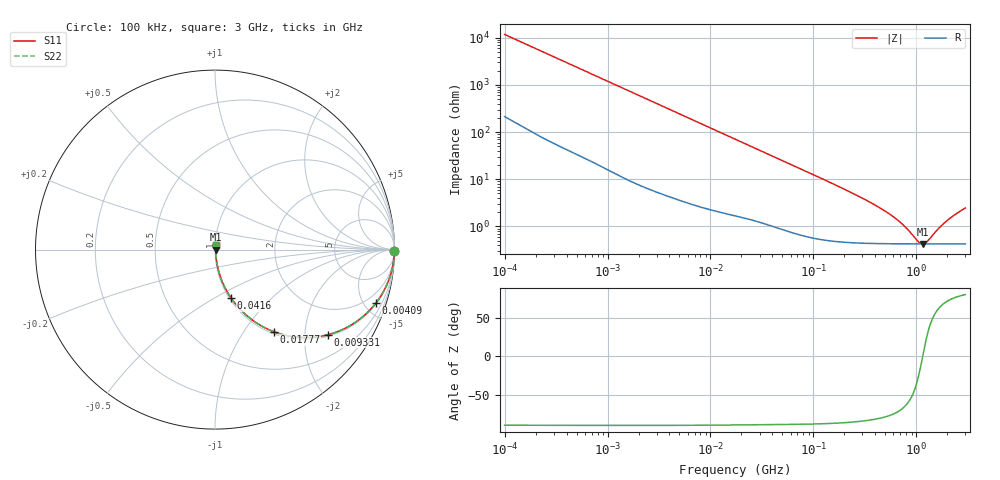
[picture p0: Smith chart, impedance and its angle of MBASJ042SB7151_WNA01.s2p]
! MBASJ042SB7151_WNA01  S-PARAMETER MODEL  ( Standard Model )
! Model Generated by TAIYO YUDEN Corporation (https://www.yuden.co.jp/en/)
! Version 1.0
! TAIYO YUDEN Control No. 250312
! Copyright(c) 2025 TAIYO YUDEN CO.,LTD. All Rights Reserved.
! Product Description (link to TY-COMPAS)
! https://ds.yuden.co.jp/TYCOMPAS/or/detail?pn=MBASJ042SB7151KWNA01&u=M
! Products Name : Multilayer Ceramic Capacitors
! Characteristics :
!  Capacitance : 150 [pF] , Rated Voltage : 6.3 [V] , TCC : X7R
!  Case Size : 0.4 x 0.2 / 0.016 x 0.008 [mm/inch] , Thickness : 0.2 / 0.008 [mm/inch]
!  (Conditions: Temperature = 25 [degC] , DC Bias Voltage = 0 [V])
! External Node Assignments :
!  1  o---| |---o  2
! GND o---------o GND
! Frequency Range : 100kHz  -  3GHz  [ 401 STEP ]
# MHZ S RI R 50
! Freq[MHz].  S11 Real  S11 Imag  S21 Real  S21 Imag  S12 Real  S12 Imag  S22 Real  S22 Imag
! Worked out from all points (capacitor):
!   401 points, 100 kHz to 3 GHz, reference 50 ohm
!   read as one part in series: C = 135 pF near 105.3 kHz
!   lowest |Z| = 425 mohm at 1.156 GHz (marker M1)
!   series resonance near 1.153 GHz, so ESL is about 140 pH
!   S11 on the Smith chart (normalised r, x): 100 kHz: open; 4.09 MHz: 1.08, -5.94; 9.331 MHz: 1.05, -2.62; 17.77 MHz: 1.03, -1.39; 41.6 MHz: 1.02, -0.60; 3 GHz: 1.01, +0.05
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0.1  0.9998 -0.00848  0.000225 0.00848  0.000225 0.00848  0.9998 -0.00848
0.562235  0.9971 -0.0467  0.00285 0.0467  0.00285 0.0467  0.9971 -0.0467
1.458987  0.9842 -0.1187  0.0158 0.1187  0.0158 0.1187  0.9842 -0.1187
3.161081  0.9337 -0.2423  0.0663 0.2423  0.0663 0.2423  0.9337 -0.2423
4.09038  0.895 -0.2997  0.105 0.2997  0.105 0.2997  0.895 -0.2997
6.178009  0.7921 -0.3981  0.2079 0.3981  0.2079 0.3981  0.7921 -0.3981
9.331111  0.63 -0.474  0.37 0.474  0.37 0.474  0.63 -0.474
12.71297  0.4825 -0.4896  0.5175 0.4896  0.5175 0.4896  0.4825 -0.4896
17.7727  0.3282 -0.4577  0.6718 0.4577  0.6718 0.4577  0.3282 -0.4577
26.84345  0.1825 -0.3723  0.8175 0.3723  0.8175 0.3723  0.1825 -0.3723
41.60216  0.0899 -0.2702  0.9101 0.2702  0.9101 0.2702  0.0899 -0.2702
97.38194  0.0217 -0.1251  0.9783 0.1251  0.9783 0.1251  0.0217 -0.1251
287.4592  0.00608 -0.0409  0.9939 0.0409  0.9939 0.0409  0.00608 -0.0409
547.5153  0.00458 -0.0178  0.9954 0.0178  0.9954 0.0178  0.00458 -0.0178
745.9503  0.00434 -0.00979  0.9957 0.00979  0.9957 0.00979  0.00434 -0.00979
1042.837  0.00424 -0.0022  0.9958 0.0022  0.9958 0.0022  0.00424 -0.0022
1156.079  0.00423 5.08e-05  0.9958 -5.08e-05  0.9958 -5.08e-05  0.00423 5.08e-05
1281.618  0.00424 0.0023  0.9958 -0.0023  0.9958 -0.0023  0.00424 0.0023
1658.39  0.0043 0.00808  0.9957 -0.00808  0.9957 -0.00808  0.0043 0.00808
1986.261  0.00438 0.0124  0.9956 -0.0124  0.9956 -0.0124  0.00438 0.0124
2504.792  0.00458 0.0186  0.9954 -0.0186  0.9954 -0.0186  0.00458 0.0186
3000  0.00481 0.0241  0.9952 -0.0241  0.9952 -0.0241  0.00481 0.0241
